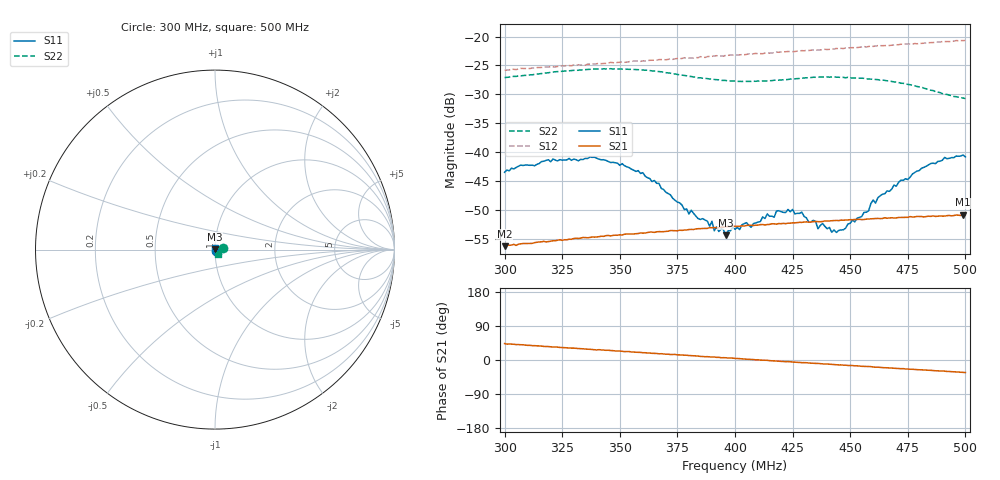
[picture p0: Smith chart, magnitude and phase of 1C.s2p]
!Prosund Technologies,SP809B,SP82221046,V.03.04.C
!Date: Monday, March 31, 2025 16:32:16
!Correction: S11(C* 2-Port  )
!S21(C* 2-Port  )
!S12(C* 2-Port  )
!S22(C* 2-Port  )
!S2P File: Measurement: :
# Hz S  dB  R 50
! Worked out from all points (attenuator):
!   201 points, 300 MHz to 500 MHz, reference 50 ohm
!   highest |S21| = -50.84 dB at 499 MHz (marker M1); lowest = -56.3 dB at 300 MHz (marker M2)
!   lowest |S11| = -54.4 dB at 396 MHz (marker M3), VSWR 1.00, Z = 49.9 + j0.174 ohm
!   |S11| at or under -10 dB: start of sweep to end of sweep
!   |S22| runs from -30.8 to -25.6 dB; largest |S21 - S12| = 0.09
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3e8  -43.50 -63.1  -56.30 43.4  -25.83 31.6  -27.10 10.6
3.21e8  -41.20 -54.4  -55.37 34.2  -25.24 28.1  -26.15 1.2
3.34e8  -41.30 -47.9  -54.80 29.7  -24.92 26.6  -25.76 -0.9
3.51e8  -42.01 -20.5  -54.38 23.0  -24.34 24.7  -25.64 -2.3
3.67e8  -45.43 5.1  -53.78 16.3  -23.99 23.0  -26.07 -3.5
3.8e8  -50.73 39.0  -53.42 11.8  -23.71 20.9  -26.90 -7.4
3.81e8  -50.08 42.3  -53.40 11.4  -23.69 21.2  -26.91 -7.7
3.89e8  -52.85 73.1  -53.09 8.3  -23.44 19.6  -27.34 -12.0
3.9e8  -51.99 85.5  -53.11 7.8  -23.43 20.0  -27.34 -12.6
3.91e8  -53.64 93.1  -53.08 7.8  -23.36 20.1  -27.44 -13.2
3.96e8  -54.43 113.2  -52.93 5.9  -23.25 19.1  -27.61 -16.0
4e8  -53.38 140.9  -52.87 4.3  -23.13 18.2  -27.72 -18.8
4.23e8  -49.94 -142.5  -52.32 -4.2  -22.59 16.0  -27.44 -31.8
4.34e8  -51.83 -121.6  -52.05 -8.5  -22.32 14.8  -27.05 -35.3
4.36e8  -53.29 -118.1  -52.05 -9.0  -22.34 14.6  -27.01 -35.4
4.38e8  -52.37 -106.0  -52.04 -10.2  -22.29 14.7  -27.01 -35.9
4.42e8  -53.90 -81.4  -51.89 -11.6  -22.18 14.2  -27.02 -36.3
4.47e8  -53.47 -48.5  -51.80 -13.7  -22.08 13.5  -27.06 -35.9
4.67e8  -46.81 34.2  -51.41 -20.9  -21.55 11.1  -27.69 -37.3
4.85e8  -41.98 65.4  -51.15 -27.2  -21.07 9.3  -29.30 -41.7
4.99e8  -40.50 84.9  -50.84 -32.6  -20.70 8.0  -30.64 -49.4
5e8  -40.86 86.4  -50.91 -33.1  -20.68 7.3  -30.75 -49.8
